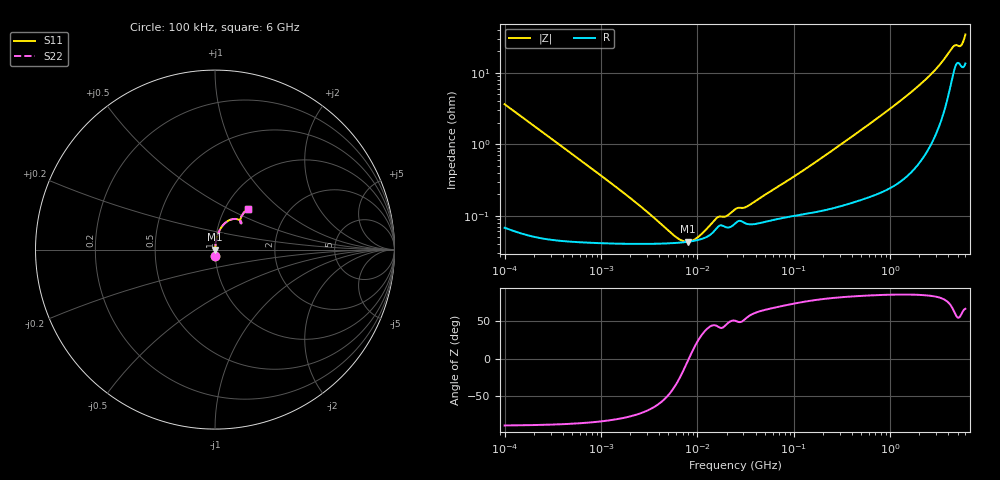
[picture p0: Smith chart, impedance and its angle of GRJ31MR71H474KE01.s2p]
!Murata Part Number: GRJ31MR71H474KE01
!These Parameters are Measured in Series Mode Connection
!Data Generated on Jun 19, 2026
!  o--ll--o
!Port1  Port2
!  o------o
!Operation Temp=25[degC], DC Bias Voltage=0[V]
!Freq. Start=100[kHz] Stop=6[GHz] 401[Steps]
# Hz S RI R 50
!Freq.(Hz) S11(Real) S11(Imag) S21(Real) S21(Imag) S12(Real) S12(Imag) S22(Real) S22(Imag)
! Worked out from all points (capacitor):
!   401 points, 100 kHz to 6 GHz, reference 50 ohm
!   read as one part in series: C = 437 nF near 105.7 kHz
!   lowest |Z| = 43.1 mohm at 7.931 MHz (marker M1)
!   series resonance near 8.124 MHz, so ESL is about 880 pH
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100000  0.00199 -0.0363  0.998 0.0363  0.998 0.0363  0.00199 -0.0363
631452  0.000456 -0.00576  0.9995 0.00576  0.9995 0.00576  0.000456 -0.00576
1950297  0.000405 -0.00178  0.9996 0.00178  0.9996 0.00178  0.000405 -0.00178
3987316  0.000405 -0.000701  0.9996 0.000701  0.9996 0.000701  0.000405 -0.000701
6191655  0.000416 -0.00025  0.9996 0.00025  0.9996 0.00025  0.000416 -0.00025
7104501  0.000423 -0.000123  0.9996 0.000123  0.9996 0.000123  0.000423 -0.000123
7930766  0.00043 -2.19e-05  0.9996 2.19e-05  0.9996 2.19e-05  0.00043 -2.19e-05
8853126  0.00044 7.92e-05  0.9996 -7.92e-05  0.9996 -7.92e-05  0.00044 7.92e-05
1.015836e7  0.000457 0.000209  0.9995 -0.000209  0.9995 -0.000209  0.000457 0.000209
1.621418e7  0.000692 0.00065  0.9993 -0.00065  0.9993 -0.00065  0.000692 0.00065
2.020496e7  0.000684 0.000722  0.9993 -0.000722  0.9993 -0.000722  0.000684 0.000722
2.517799e7  0.0008 0.000966  0.9992 -0.000966  0.9992 -0.000966  0.0008 0.000966
3.407377e7  0.000758 0.00116  0.9992 -0.00116  0.9992 -0.00116  0.000758 0.00116
1.546735e8  0.00112 0.00509  0.9989 -0.00509  0.9989 -0.00509  0.00112 0.00509
9.76689e8  0.00333 0.0307  0.9967 -0.0307  0.9967 -0.0307  0.00333 0.0307
1.942633e9  0.0093 0.0639  0.9907 -0.0639  0.9907 -0.0639  0.0093 0.0639
3.100717e9  0.0291 0.1143  0.9709 -0.1143  0.9709 -0.1143  0.0291 0.1143
3.759065e9  0.0575 0.1493  0.9425 -0.1493  0.9425 -0.1493  0.0575 0.1493
4.433555e9  0.1154 0.1708  0.8846 -0.1708  0.8846 -0.1708  0.1154 0.1708
4.814911e9  0.1448 0.1563  0.8552 -0.1563  0.8552 -0.1563  0.1448 0.1563
5.374892e9  0.1402 0.1554  0.8598 -0.1554  0.8598 -0.1554  0.1402 0.1554
6e9  0.1831 0.2283  0.8169 -0.2283  0.8169 -0.2283  0.1831 0.2283
